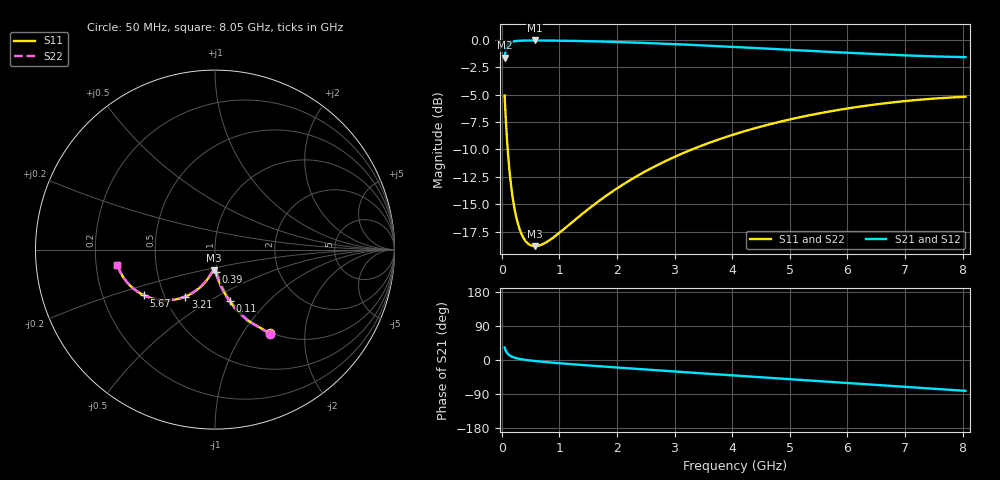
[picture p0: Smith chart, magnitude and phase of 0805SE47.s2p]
! AVX Thin Film Operation		Date: August 2001
! Description: Accu-P® Series, Thin Film, SMD, RF Capacitor
! Part Number: 08053K470FBT
! 50 MHz  -  8.05 GHz
! Serial Measurements
# mhz S db R 50
!	S11		S21		S12		S22
!	dB	Phase	dB	Phase	dB	Phase	dB	Phase
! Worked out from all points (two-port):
!   401 points, 50 MHz to 8.05 GHz, reference 50 ohm
!   highest |S21| = -0.06 dB at 570 MHz (marker M1); lowest = -1.6 dB at 50 MHz (marker M2)
!   |S21| within 3 dB of the highest: start of sweep to end of sweep
!   lowest |S11| = -18.8 dB at 570 MHz (marker M3), VSWR 1.26, Z = 48.3 - j11.2 ohm
!   |S11| at or under -10 dB: 103.7 MHz to 3.303 GHz (3.199 GHz wide, 188 % of centre)
!   |S22| runs from -18.8 to -5.1 dB; largest |S21 - S12| = 0
!   S11 on the Smith chart (normalised r, x): 50 MHz: 0.98, -1.33; 110 MHz: 0.98, -0.62; 390 MHz: 0.98, -0.24; 3.21 GHz: 0.63, -0.37; 5.67 GHz: 0.39, -0.25; 8.05 GHz: 0.29, -0.07
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50  -5.07 -56.8  -1.62 33.1  -1.62 33.1  -5.07 -57.0
70  -7.21 -65.1  -0.92 24.7  -0.92 24.7  -7.21 -65.4
110  -10.47 -74.1  -0.41 15.7  -0.41 15.7  -10.47 -74.4
130  -11.69 -76.8  -0.31 13.0  -0.31 13.0  -11.69 -77.1
170  -13.62 -80.4  -0.20 9.3  -0.20 9.3  -13.62 -80.9
230  -15.62 -83.8  -0.12 5.8  -0.12 5.8  -15.62 -84.4
310  -17.26 -86.6  -0.09 2.9  -0.09 2.9  -17.26 -87.4
390  -18.17 -88.6  -0.07 0.8  -0.07 0.8  -18.17 -89.5
470  -18.64 -90.3  -0.06 -0.8  -0.06 -0.8  -18.64 -91.1
570  -18.82 -92.0  -0.06 -2.6  -0.06 -2.6  -18.82 -92.9
830  -18.28 -95.8  -0.07 -6.3  -0.07 -6.3  -18.28 -96.6
1390  -15.91 -102.6  -0.12 -13.1  -0.12 -13.1  -15.91 -103.3
2050  -13.38 -110.0  -0.21 -20.3  -0.21 -20.3  -13.38 -110.4
2730  -11.35 -117.2  -0.34 -27.5  -0.34 -27.5  -11.35 -117.6
3210  -10.20 -122.2  -0.44 -32.5  -0.44 -32.5  -10.20 -122.5
4050  -8.60 -130.8  -0.65 -41.1  -0.65 -41.1  -8.60 -131.0
4730  -7.60 -137.7  -0.84 -47.9  -0.84 -47.9  -7.60 -137.9
5390  -6.83 -144.3  -1.02 -54.5  -1.02 -54.5  -6.83 -144.4
5670  -6.55 -147.1  -1.10 -57.3  -1.10 -57.3  -6.55 -147.2
6730  -5.74 -157.7  -1.36 -67.9  -1.36 -67.9  -5.74 -157.8
7430  -5.39 -164.8  -1.50 -75.0  -1.50 -75.0  -5.39 -164.8
8050  -5.20 -171.2  -1.58 -81.4  -1.58 -81.4  -5.20 -171.3
